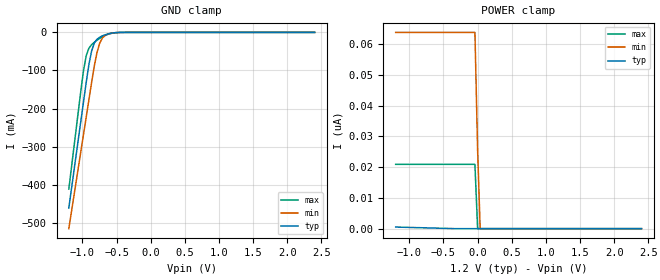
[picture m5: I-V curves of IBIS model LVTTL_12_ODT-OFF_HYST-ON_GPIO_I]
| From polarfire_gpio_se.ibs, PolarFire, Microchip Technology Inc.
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|   Model LVTTL_12_ODT-OFF_HYST-ON_GPIO_I
[Model]   LVTTL_12_ODT-OFF_HYST-ON_GPIO_I
Model_type   Input
Vinl =   0.8
Vinh =   2.0
|   typ   min   max
C_comp_pullup   2.605e-12   2.605e-12   2.76e-12
C_comp_pulldown  2.605e-12   2.605e-12   2.76e-12
[Model Spec]
Vinh+   1.733   1.654   1.811
Vinh-   1.733   1.654   1.811
Vinl+   1.568   1.496   1.639
Vinl-   1.568   1.496   1.639
[Temperature Range]  25C   100C   -40C
[Voltage Range]  1.2   1.14   1.26
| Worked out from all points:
|   GND clamp passes 1 mA (typ) near -0.53 V on its own axis
[GND Clamp]
| Voltage   I(typ)   I(min)   I(max)
-1.2V     -460.9mA   -515.3mA   -411.5mA
-1.024V   -232.8mA   -312.7mA   -153.3mA
-984.4mV  -181.9mA   -267.4mA   -99.94mA
-945mV    -131.1mA   -222.2mA   -61.15mA
-905.6mV  -84.23mA   -176.9mA   -41.34mA
-866.2mV  -48.93mA   -131.7mA   -32.26mA
-826.9mV  -28.05mA   -88.35mA   -26.02mA
-787.5mV  -17.96mA   -52.99mA   -20.61mA
-748.1mV  -12.65mA   -28.64mA   -15.79mA
-669.4mV  -6.309mA   -8.083mA   -8.082mA
-433.1mV  -82.31uA   -116.2uA   -108.2uA
2.4V      0A         0A         0A
[POWER Clamp]
| Voltage   I(typ)   I(min)   I(max)
-1.2V     519.2pA    63.89nA    20.93nA
-39.38mV  -1.999pA   63.89nA    20.93nA
0V        0A         25.56nA    0A
37.5mV    0A         0A         0A
2.4V      0A         0A         0A
